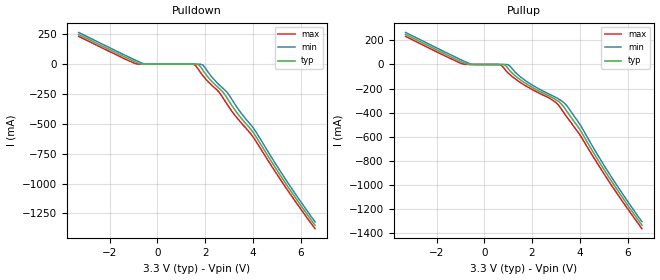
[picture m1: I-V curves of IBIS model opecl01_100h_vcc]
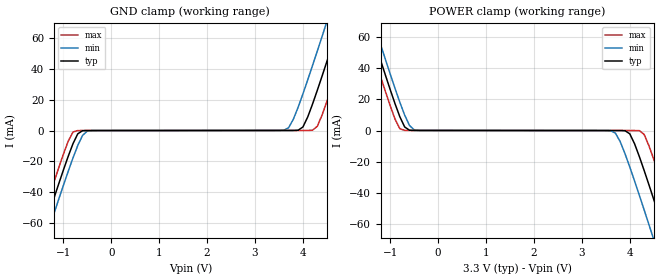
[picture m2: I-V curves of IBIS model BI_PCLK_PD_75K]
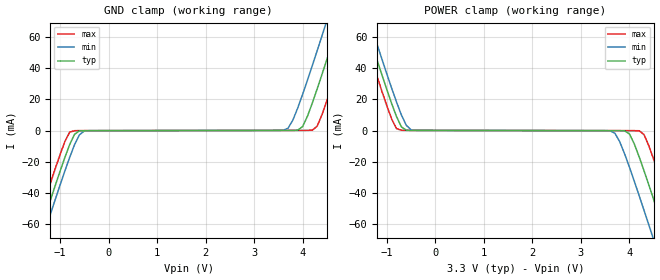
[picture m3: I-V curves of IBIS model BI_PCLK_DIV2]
|   This file is an IBIS representation of the   |
|   Integrated Device Technology   |
|   ICS853111A-02   |
|   Low Skew 1 to 10 LVPECL Clock Buffer   |
[IBIS Ver]   3.2
[File name]   853111a-02_3v3.ibs
[File Rev]   1.0
[Date]   May 29 2007 | Last modified
|   May 29 2007 | Generated
[Source] Originated at Integrated Device Technology.
[Disclaimer]
IDT hereby grants the user of this IBIS model a non-exclusive,
nontransferable license to use this IBIS model under the following terms.
Before using this IBIS model, the user should read this license.
If the user does not accept these terms,  the IBIS model should be
returned to IDT within 30 days.
   The user is granted this license only to use the IBIS model and
is not granted rights to sell, load, rent, lease or license the IBIS
model in whole or in part, or in modified form to anyone other than
user. User may modify the IBIS model to suit its specific
applications but rights to derivative works and such modifications
shall belong to IDT.
   This IBIS model is provided on an "AS IS" basis and IDT makes
absolutely no warranty with respect to the information contained
herein. IDT DISCLAIMS AND CUSTOMER WAIVES ALL WARRANTIES, EXPRESS
OR IMPLIED, INCLUDING WARRANTIES OF MERCHANTABILITY OR FITNESS FOR
A PARTICULAR PURPOSE. The entire risk as to quality and performance
is with the Customer. ACCORDINGLY, IN NO EVENT SHALL THE COMPANY BE
LIABLE FOR ANY DAMAGES, WHETHER IN CONTRACT OR TORT,INCLUDING ANY
LOST PROFITS OR OTHER INCIDENTAL, CONSEQUENTIAL, EXEMPLARY, OR
PUNITIVE DAMAGES ARISING OUT OF THE USE OR APPLICATION OF THE IBIS
model provided in this package. Further, IDT reserves the right to
make changes without notice to any product herein to improve
reliability, function, or design. IDT does not convey any license
under patent rights or any other intellectual property rights,
including those of third parties.
   IDT is not obligated to provide maintenance or support
for the licensed IBIS model.
[Copyright]   Copyright 2007 by Integrated Device Technology.
[Component]   ICS853111A-02
[Manufacturer] Integrated Device Technology.
[Package]
|TQFP32
|lead + wire   typ   min   max
R_pkg   58.4m   52.7m   64.1m
L_pkg   2.197nH   1.997nH   2.397n
C_pkg   0.267pF   0.255pF   0.278pF
[Pin] signal_name   model_name
1   VCC   POWER
2   CLK_SEL   BI_INPUT_PD
3   PCLK0   BI_PCLK_PD_75K
4   nPCLK0   BI_PCLK_DIV2
|5   VBB
6   PCLK1   BI_PCLK_PD_75K
7   nPCLK1   BI_PCLK_DIV2
8   VEE   GND
9   VCCO   POWER
10   nQ9   opecl01_100h_vcc
11   Q9   opecl01_100h_vcc
12   nQ8   opecl01_100h_vcc
13   Q8   opecl01_100h_vcc
14   nQ7   opecl01_100h_vcc
15   Q7   opecl01_100h_vcc
16   VCCO   POWER
17   nQ6   opecl01_100h_vcc
18   Q6   opecl01_100h_vcc
19   nQ5   opecl01_100h_vcc
20   Q5   opecl01_100h_vcc
21   nQ4   opecl01_100h_vcc
22   Q4   opecl01_100h_vcc
23   nQ3   opecl01_100h_vcc
24   Q3   opecl01_100h_vcc
25   VCCO   POWER
26   nQ2   opecl01_100h_vcc
27   Q2   opecl01_100h_vcc
28   nQ1   opecl01_100h_vcc
29   Q1   opecl01_100h_vcc
30   nQ0   opecl01_100h_vcc
31   Q0   opecl01_100h_vcc
32   VCCO   POWER
[Diff Pin]  inv_pin  vdiff tdelay_typ tdelay_min  tdelay_max
11   10   NA   0  0  0
13   12   NA   0  0  0
15   14   NA   0  0  0
18   17   NA   0  0  0
20   19   NA   0  0  0
22   21   NA   0  0  0
24   23   NA   0  0  0
27   26   NA   0  0  0
29   28   NA   0  0  0
31   30   NA   0  0  0
| Models and submodels in the file (4): opecl01_100h_vcc (Output_ECL), BI_PCLK_PD_75K (Input_ECL), BI_PCLK_DIV2 (Input), BI_INPUT_PD (Input)
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[Model]   opecl01_100h_vcc
Model_type  Output_ECL
Polarity   Non-Inverting
|Variable   typ   min   max
C_comp   2p   1.5p  2.5p
|Variable   typ   min   max
[Temperature Range]   25   85   -40
[Voltage Range]   3.3   3.135   3.465
|  Voltage   I(typ)   I(min)   I(max)
[Pullup]
-3.3V     250.2mA    266.5mA    233.9mA
-900mV    17.14mA    32.04mA    4.25mA
-500mV    2.485uA    997.2uA    4.222nA
700mV     -10.62uA   -20.41nA   -4.03mA
900mV     -9.721mA   -40.89uA   -50.21mA
1V        -34.71mA   -1.618mA   -70.69mA
1.8V      -165.5mA   -144.4mA   -185.1mA
2.9V      -281.1mA   -264mA     -301.8mA
3.3V      -345.3mA   -311.8mA   -391.8mA
4V        -540.3mA   -496.2mA   -583.4mA
5.2V      -931.2mA   -896.4mA   -965.2mA
6.6V      -1.335A    -1.306A    -1.364A
[Pulldown]
-3.3V     250.2mA    266.5mA    233.9mA
-1V       26.06mA    41.37mA    11.64mA
-500mV    2.485uA    997.2uA    4.222nA
1.5V      -1.258uA   -2.492nA   -603.5uA
1.7V      -2.133mA   -5.026uA   -38.67mA
1.9V      -49.4mA    -6.147mA   -94.61mA
2.6V      -205.2mA   -175.7mA   -238.5mA
2.9V      -278.7mA   -231.3mA   -330.4mA
3.4V      -425.4mA   -380.9mA   -466.1mA
4V        -568.5mA   -530.2mA   -607.1mA
5.4V      -1.008A    -974.4mA   -1.041A
6.6V      -1.35A     -1.321A    -1.378A
[Ramp]
|   typ   min   max
dV/dt_r   0.48V/0.20ns   0.48V/0.25ns   0.48V/0.15ns
dV/dt_f   0.48V/0.20ns   0.48V/0.25ns   0.48V/0.15ns
R_load =   50.0000
[Model]   BI_PCLK_PD_75K
Model_type   Input_ECL
Polarity   Non-Inverting
Vinl = 1.825V
Vinh = 2.135V
|   typ   min   max
C_comp   2pF   1.5pF   2.5pF
|   typ   min   max
[Voltage range]  3.3V   3.15V   3.45V
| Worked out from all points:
|   GND clamp passes 1 mA (typ) near -0.64 V on its own axis
|   POWER clamp passes 1 mA (typ) near -0.64 V on its own axis
[GND_clamp]
| |Voltage I(typ)   I(min)   I(max)
-3.3V     -249.9mA   -259.6mA   -239.9mA
-1.5V     -73.07mA   -83.13mA   -62.6mA
-1.3V     -53.85mA   -63.93mA   -43.34mA
-700mV    -2.138mA   -9.736mA   -18.88uA
-400mV    -5.182uA   -19.02uA   -4.67uA
3.6V      50.33uA    175uA      46.37uA
4V        2.304mA    23.88mA    51.37uA
4.2V      17.18mA    42.31mA    198.2uA
4.5V      44.99mA    71mA       18.95mA
4.7V      64.27mA    90.46mA    37.76mA
5V        93.61mA    119.9mA    66.91mA
6.6V      252.7mA    278.9mA    226.1mA
[POWER_clamp]
|Voltage   I(typ)   I(min)   I(max)
-3.3V     252.7mA    262.5mA    242.7mA
-1.6V     83.79mA    93.88mA    73.29mA
-1.4V     64.27mA    74.39mA    53.71mA
-700mV    2.305mA    9.955mA    121.2uA
-400mV    51.76uA    67.82uA    49.5uA
3.6V      -3.857uA   -114.5uA   -1.576uA
4V        -2.14mA    -23.52mA   -6.249uA
4.2V      -16.83mA   -41.74mA   -68.23uA
4.5V      -44.35mA   -70.15mA   -18.54mA
4.7V      -63.43mA   -89.4mA    -37.15mA
5V        -92.47mA   -118.5mA   -66mA
6.6V      -249.9mA   -275.9mA   -223.6mA
[Model]   BI_PCLK_DIV2
Model_type   Input
Polarity   Non-Inverting
Vinl = 0.70V
Vinh = 0.88V
|   typ   min   max
C_comp   2pF   1.5pF   2.5pF
|   typ   min   max
[Voltage range]  3.3V   3.15V   3.45V
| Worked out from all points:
|   GND clamp passes 1 mA (typ) near -0.64 V on its own axis
|   POWER clamp passes 1 mA (typ) near -0.64 V on its own axis
[GND_clamp]
|Voltage   I(typ)   I(min)   I(max)
-3.3V     -250.4mA   -259mA     -240.1mA
-1.6V     -83.18mA   -92.05mA   -72.41mA
-1.4V     -63.86mA   -72.75mA   -53.03mA
-700mV    -2.406mA   -9.083mA   -95.91uA
-400mV    -79.29uA   -88.9uA    -74.69uA
3.6V      79.42uA    173uA      69.75uA
4V        2.532mA    23.1mA     84.09uA
4.2V      17.54mA    41.5mA     235.6uA
4.5V      45.37mA    70.2mA     19mA
4.7V      64.66mA    89.67mA    37.81mA
5V        94.01mA    119.1mA    66.96mA
6.6V      253.2mA    278.2mA    226.2mA
[POWER_clamp]
|Voltage   I(typ)   I(min)   I(max)
-3.3V     252.8mA    262.6mA    242.8mA
-1.6V     83.86mA    93.94mA    73.35mA
-1.4V     64.33mA    74.45mA    53.77mA
-700mV    2.344mA    9.996mA    157.8uA
-400mV    83.25uA    99.97uA    79.07uA
3.6V      -75.19uA   -191uA     -65.41uA
4V        -2.222mA   -23.6mA    -79.43uA
4.2V      -16.92mA   -41.84mA   -146.1uA
4.5V      -44.44mA   -70.25mA   -18.63mA
4.7V      -63.53mA   -89.51mA   -37.24mA
5V        -92.57mA   -118.7mA   -66.09mA
6.6V      -250.1mA   -276.1mA   -223.7mA
